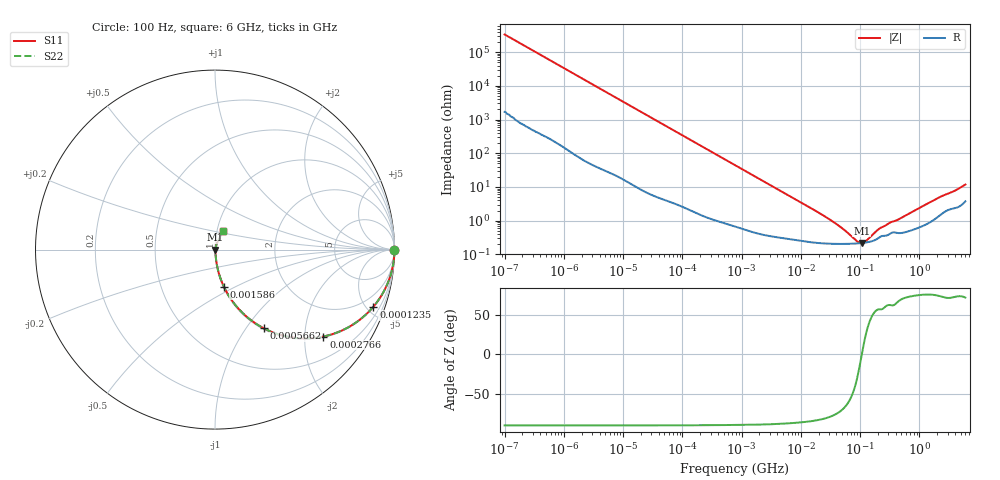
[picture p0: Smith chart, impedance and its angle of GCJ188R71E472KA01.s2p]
!Murata Part Number: GCJ188R71E472KA01
!These Parameters are Measured in Series Mode Connection
!Data Generated on Mar 13, 2026
!  o--ll--o
!Port1  Port2
!  o------o
!Operation Temp=25[degC], DC Bias Voltage=0[V]
!Freq. Start=100[Hz] Stop=6[GHz] 401[Steps]
# Hz S RI R 50
!Freq.(Hz) S11(Real) S11(Imag) S21(Real) S21(Imag) S12(Real) S12(Imag) S22(Real) S22(Imag)
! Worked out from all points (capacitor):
!   401 points, 100 Hz to 6 GHz, reference 50 ohm
!   read as one part in series: C = 4.75 nF near 109 Hz
!   lowest |Z| = 217 mohm at 106.7 MHz (marker M1)
!   series resonance near 107.1 MHz, so ESL is about 460 pH
!   S11 on the Smith chart (normalised r, x): 100 Hz: open; 123.5 kHz: 1.04, -5.53; 276.6 kHz: 1.02, -2.48; 566.2 kHz: 1.02, -1.21; 1.586 MHz: 1.01, -0.44; 6 GHz: 1.08, +0.22
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100  1 -0.000299  1.6e-06 0.000299  1.6e-06 0.000299  1 -0.000299
2008  0.9999 -0.00596  5.91e-05 0.00596  5.91e-05 0.00596  0.9999 -0.00596
12592  0.9984 -0.0371  0.00156 0.0371  0.00156 0.0371  0.9984 -0.0371
40335  0.9855 -0.1169  0.0145 0.1169  0.0145 0.1169  0.9855 -0.1169
123542  0.8823 -0.3183  0.1177 0.3183  0.1177 0.3183  0.8823 -0.3183
184852  0.772 -0.4153  0.228 0.4153  0.228 0.4153  0.772 -0.4153
276587  0.6045 -0.4842  0.3955 0.4842  0.3955 0.4842  0.6045 -0.4842
395726  0.43 -0.4895  0.57 0.4895  0.57 0.4895  0.43 -0.4895
566185  0.2722 -0.4386  0.7278 0.4386  0.7278 0.4386  0.2722 -0.4386
774597  0.169 -0.3673  0.831 0.3673  0.831 0.3673  0.169 -0.3673
1585629  0.0494 -0.2067  0.9506 0.2067  0.9506 0.2067  0.0494 -0.2067
4246196  0.00978 -0.081  0.9902 0.081  0.9902 0.081  0.00978 -0.081
1.555665e7  0.00276 -0.0222  0.9972 0.0222  0.9972 0.0222  0.00276 -0.0222
4.165952e7  0.00209 -0.00725  0.9979 0.00725  0.9979 0.00725  0.00209 -0.00725
8.918374e7  0.00211 -0.00123  0.9979 0.00123  0.9979 0.00123  0.00211 -0.00123
1.066761e8  0.00217 -2.9e-05  0.9978 2.9e-05  0.9978 2.9e-05  0.00217 -2.9e-05
1.275994e8  0.00226 0.00118  0.9977 -0.00118  0.9977 -0.00118  0.00226 0.00118
2.088084e8  0.00314 0.00475  0.9969 -0.00475  0.9969 -0.00475  0.00314 0.00475
3.124326e8  0.00401 0.00748  0.996 -0.00748  0.996 -0.00748  0.00401 0.00748
4.470121e8  0.00436 0.01  0.9956 -0.01  0.9956 -0.01  0.00436 0.01
2.048624e9  0.0146 0.0437  0.9854 -0.0437  0.9854 -0.0437  0.0146 0.0437
6e9  0.0473 0.1031  0.9527 -0.1031  0.9527 -0.1031  0.0473 0.1031
